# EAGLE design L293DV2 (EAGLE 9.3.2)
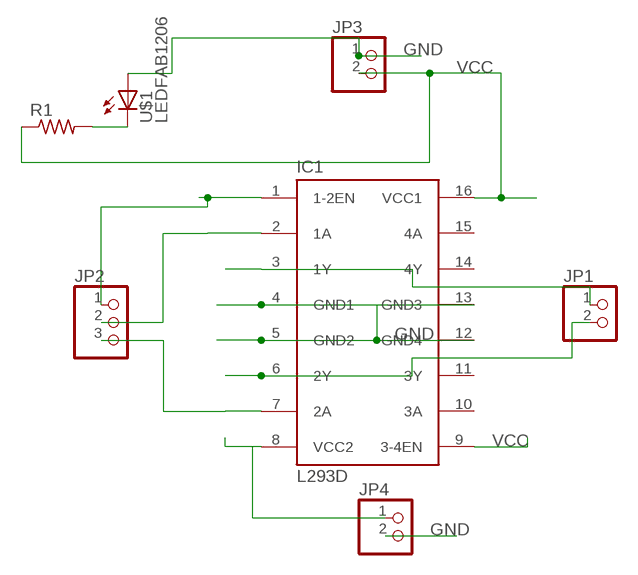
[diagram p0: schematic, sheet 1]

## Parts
IC1  L293D  [DIL16]
JP1  PINHD-1X2  [1X02]
JP2  PINHD-1X3  [1X03]
JP3  PINHD-1X2  [1X02]
JP4  PINHD-1X2  [1X02]
R1  RES-US1206FAB  [R1206FAB]
U$1  LEDFAB1206  [LED1206FAB]

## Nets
GND: IC1.4(GND1) IC1.5(GND2) IC1.12(GND4) IC1.13(GND3) JP3.1 JP4.2 U$1.1(A)
N$1: IC1.1(1-2EN) JP2.1
N$2: IC1.2(1A) JP2.2
N$3: IC1.3(1Y) JP1.1
N$4: R1.2 U$1.2(C)
N$6: IC1.6(2Y) JP1.2
N$7: IC1.8(VCC2) JP4.1
N$8: IC1.7(2A) JP2.3
VCC: IC1.9(3-4EN) IC1.16(VCC1) JP3.2 R1.1
Unconnected: IC1.10(3A) IC1.11(3Y) IC1.14(4Y) IC1.15(4A)

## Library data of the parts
IC1 = st-microelectronics:L293D: PUSH-PULL 4 CHANNEL DRIVER; MPN: L293D; OC_FARNELL: 9589619; OC_NEWARK: 56P8249
JP1 JP3 JP4 = pinhead:PINHD-1X2: PIN HEADER
JP2 = pinhead:PINHD-1X3: PIN HEADER
R1 = fab:RES-US: Resistor (US Symbol)
U$1 = fab:LED: LED

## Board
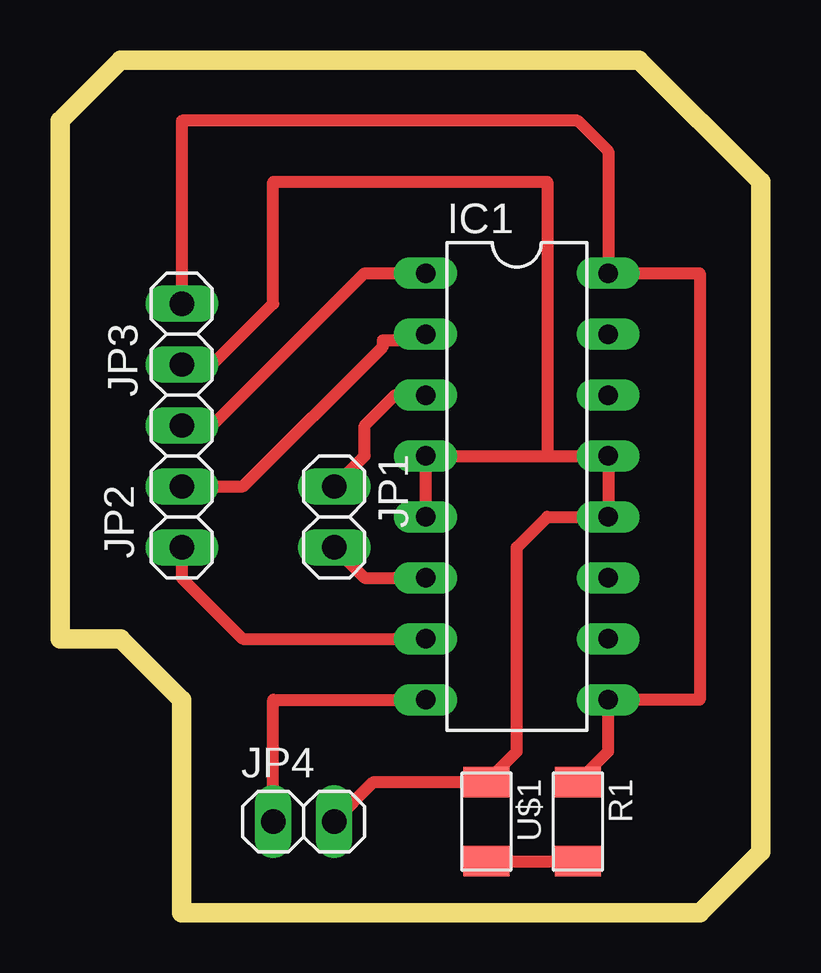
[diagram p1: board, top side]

Size 29.21 x 35.56 mm. Coordinates in mm from the lower left corner, seen from the top.
Outline: 0,33.02 0,11.43 2.54,11.43 5.08,8.89 5.08,0 26.67,0 29.21,2.54 29.21,30.48 24.13,35.56 2.54,35.56 0,33.02
Copper layers (1*16): Top 0.035mm / dielectric 1.5mm / Bottom 0.035mm
Design rules "default": minimum track width 6mil, minimum drill 0.35mm, track to track 6mil, track to pad 6mil, pad to pad 6mil, via to via 6mil, smd to smd 6mil, copper to edge 40mil, drill to drill 6mil, minimum pad ring 10mil, minimum via ring 8mil, stop-mask expansion 4mil, vias tented up to drill 0mil, thermal gap 10mil

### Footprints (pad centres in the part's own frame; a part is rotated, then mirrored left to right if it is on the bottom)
DIL16 = drill 0.813 long: 1 -8.89,-3.81; 2 -6.35,-3.81; 3 -3.81,-3.81; 4 -1.27,-3.81; 5 1.27,-3.81; 6 3.81,-3.81; 7 6.35,-3.81; 8 8.89,-3.81; 9 8.89,3.81; 10 6.35,3.81; 11 3.81,3.81; 12 1.27,3.81; 13 -1.27,3.81; 14 -3.81,3.81; 15 -6.35,3.81; 16 -8.89,3.81
1X02 = drill 1.016 long: 1 -1.27,0; 2 1.27,0
1X03 = drill 1.016 long: 1 -2.54,0; 2 0,0; 3 2.54,0
R1206FAB = smd 1.27 x 1.905: 1 -1.651,0; 2 1.651,0
LED1206FAB = smd 1.27 x 1.905: 1 -1.651,0; 2 1.651,0

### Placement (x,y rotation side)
IC1  19.05,17.78 270 top
JP1  11.43,16.51 270 top
JP2  5.08,17.78 270 top
JP3  5.08,24.13 90 top
JP4  10.16,3.81 0 top
R1  21.59,3.81 270 top
U$1  17.78,3.81 270 top

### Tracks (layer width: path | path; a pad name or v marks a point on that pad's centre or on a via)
GND
  Top 0.508: 20.32,19.05 20.32,30.48 8.89,30.48 8.89,25.4 6.35,22.86 JP3.1 | 20.32,19.05 IC1.13 IC1.12 20.32,16.51 19.05,15.24 19.05,6.73 U$1.1 13.08,5.46 JP4.2 | 20.32,19.05 IC1.4 IC1.5
N$1
  Top 0.508: JP2.1 6.35,20.32 12.7,26.67 IC1.1
N$2
  Top 0.508: JP2.2 7.62,17.78 13.46,23.62 13.46,23.88 14.99,23.88 IC1.2
N$3
  Top 0.508: JP1.1 12.7,19.05 12.7,20.32 13.97,21.59 IC1.3
N$4
  Top 0.508: U$1.2 R1.2
N$6
  Top 0.508: 13.97,13.97 IC1.6 12.7,13.97 JP1.2
N$7
  Top 0.508: JP4.1 8.89,8.89 IC1.8
N$8
  Top 0.508: JP2.3 5.08,13.97 7.62,11.43 IC1.7
VCC
  Top 0.508: JP3.2 5.08,33.02 21.59,33.02 22.86,31.75 IC1.16 26.67,26.67 26.67,8.89 IC1.9 22.86,6.73 R1.1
